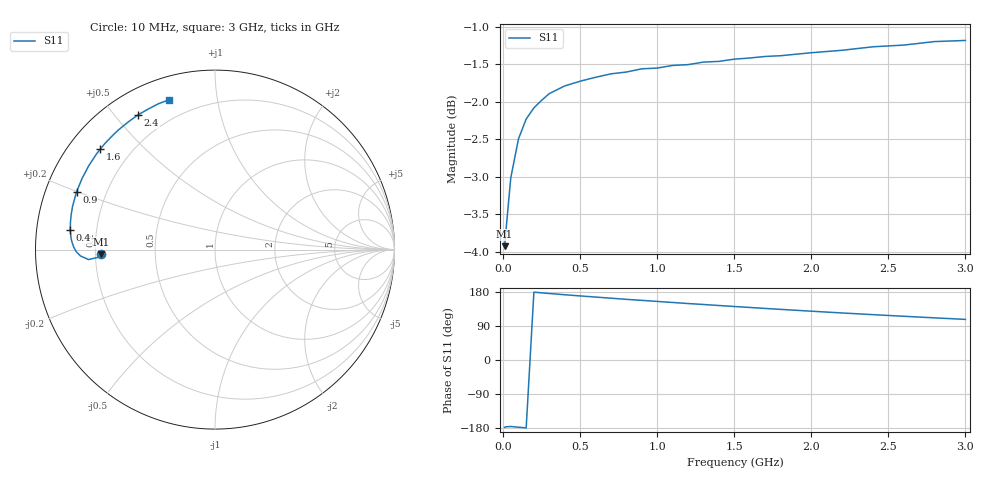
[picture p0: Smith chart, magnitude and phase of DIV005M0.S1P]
! SIEMENS Small Signal Semiconductors
! BAV99
! Silicon Switching Diode in SOT23
! IF = 5 mA
! S-Parameters:  May  1995
# GHz  S  MA  R  50
!  f  S11
! GHz  MAG  ANG
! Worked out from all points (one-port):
!   30 points, 10 MHz to 3 GHz, reference 50 ohm
!   lowest |S11| = -3.9 dB at 10 MHz (marker M1), VSWR 4.50, Z = 11.1 - j0.996 ohm
!   |S11| at or under -10 dB: nowhere
!   S11 on the Smith chart (normalised r, x): 10 MHz: 0.22, -0.02; 400 MHz: 0.10, +0.07; 900 MHz: 0.09, +0.20; 1.6 GHz: 0.09, +0.37; 2.4 GHz: 0.10, +0.58; 3 GHz: 0.10, +0.73
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0.01  0.6363 -177.6
0.02  0.6538 -176.2
0.05  0.7067 -175.5
0.1  0.7504 -177.3
0.15  0.7737 -179.2
0.2  0.7871 179.0
0.25  0.7963 177.3
0.3  0.8045 175.5
0.4  0.8141 172.2
0.5  0.82 169.1
0.6  0.825 166.1
0.7  0.8294 163.1
0.8  0.8317 160.1
0.9  0.8358 157.4
1.1  0.8401 151.8
1.2  0.8412 149.0
1.3  0.8445 146.5
1.5  0.8483 141.2
1.6  0.8498 138.7
1.7  0.8518 136.1
1.8  0.8528 133.6
1.9  0.8548 131.2
2  0.8567 128.8
2.2  0.86 124.1
2.4  0.8646 119.7
2.6  0.8669 115.4
2.8  0.8716 111.2
3  0.8731 107.2
